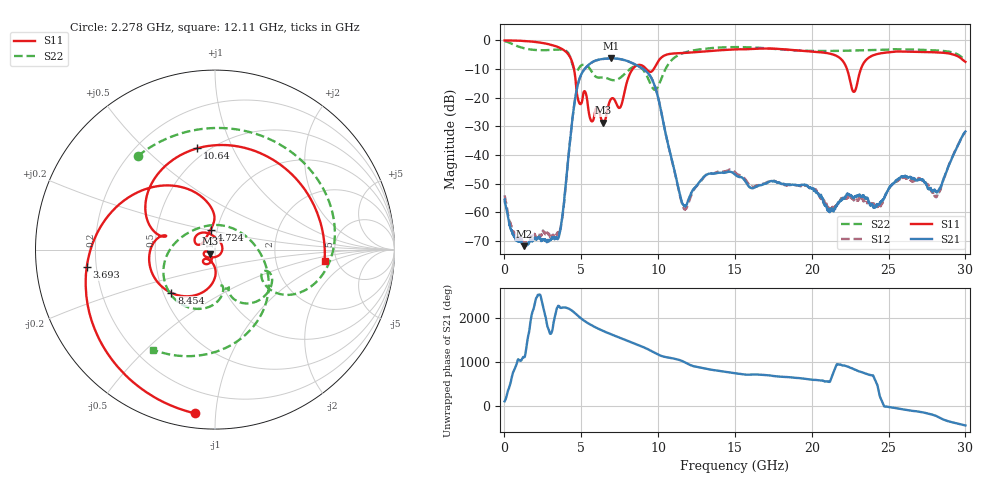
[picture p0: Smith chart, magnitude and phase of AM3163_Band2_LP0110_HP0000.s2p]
!Agilent Technologies,E8364B,MY43040894,A.07.50.67
!Agilent E8364B: A.07.50.67
!Date: Thursday, August 20, 2020 12:05:15
!Correction: S11(Full 2 Port(1,2))
!S21(Full 2 Port(1,2))
!S12(Full 2 Port(1,2))
!S22(Full 2 Port(1,2))
!S2P File: Measurements: S11, S21, S12, S22:
# Hz S  dB  R 50
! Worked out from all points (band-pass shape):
!   3201 points, 10 MHz to 30 GHz, reference 50 ohm
!   highest |S21| = -6.27 dB at 6.945 GHz (marker M1); lowest = -71.8 dB at 1.285 GHz (marker M2)
!   |S21| within 3 dB of the highest: 5.334 GHz to 8.814 GHz (3.48 GHz wide, 49.2 % of centre)
!   lowest |S11| = -28.7 dB at 6.43 GHz (marker M3), VSWR 1.08, Z = 47.1 - j2.1 ohm
!   |S11| at or under -10 dB: 4.526 GHz to 8.342 GHz (3.815 GHz wide, 59.3 % of centre); 9.234 GHz to 9.716 GHz (482 MHz wide, 5.09 % of centre); 22.29 GHz to 23.2 GHz (903.4 MHz wide, 3.97 % of centre)
!   |S22| runs from -17.3 to -0.2 dB; largest |S21 - S12| = 0.0036
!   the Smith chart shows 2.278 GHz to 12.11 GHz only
!   S11 on the Smith chart (normalised r, x): 2.278 GHz: 0.07, -0.88; 3.693 GHz: 0.16, -0.07; 4.724 GHz: 0.93, +0.21; 8.454 GHz: 0.55, -0.30; 10.64 GHz: 0.44, +0.74; 12.11 GHz: 4.01, -0.79
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1e7  -0.02 -2.9  -55.59 107.6  -54.04 -57.6  -0.24 -10.1
5.910562e8  -0.06 -24.3  -67.90 69.9  -66.82 19.2  -1.47 -80.2
1.284575e9  -0.19 -53.4  -71.80 29.9  -70.64 79.5  -2.74 -152.0
2.277994e9  -0.73 -96.9  -68.64 18.9  -68.05 -25.2  -3.41 129.6
3.693147e9  -2.83 -172.1  -64.03 74.1  -64.16 42.7  -3.20 27.6
4.724053e9  -18.83 101.9  -16.63 -86.5  -16.65 -86.8  -10.57 -24.2
5.014581e9  -21.85 154.7  -11.69 -173.1  -11.69 -173.4  -8.68 -30.8
5.530034e9  -26.29 46.2  -8.29 67.4  -8.32 67.2  -9.68 -64.2
6.429734e9  -28.70 -142.8  -6.46 -90.6  -6.47 -90.7  -12.89 -73.2
6.945188e9  -20.40 -121.8  -6.27 -166.8  -6.27 -166.8  -13.75 -80.0
7.65745e9  -21.74 -96.7  -6.65 93.7  -6.68 93.6  -12.52 -79.1
8.454059e9  -9.31 -135.1  -8.25 -15.2  -8.26 -15.1  -9.08 -111.8
1.000979e10  -7.25 152.7  -20.14 92.1  -20.04 91.5  -15.99 45.4
1.063771e10  -4.84 100.0  -36.01 26.1  -36.06 24.0  -8.54 -37.2
1.210909e10  -4.24 -5.8  -53.82 -148.0  -54.69 -149.6  -3.67 -121.6
1.5005e10  -3.15 -142.8  -46.88 24.4  -45.95 23.4  -2.32 135.3
1.771347e10  -2.93 94.4  -49.49 -42.8  -49.42 -44.0  -3.04 32.2
2.000958e10  -3.92 -26.9  -51.74 -120.7  -51.84 -120.6  -3.66 -49.8
2.274617e10  -17.96 -109.7  -55.03 119.3  -55.75 115.4  -3.52 -127.5
2.500479e10  -4.17 -151.4  -51.69 -20.5  -52.16 -23.8  -3.23 176.8
2.814437e10  -4.17 109.0  -52.99 124.9  -54.46 118.9  -3.48 92.4
3e10  -7.47 38.4  -31.78 -81.4  -32.05 -78.3  -6.92 35.2
